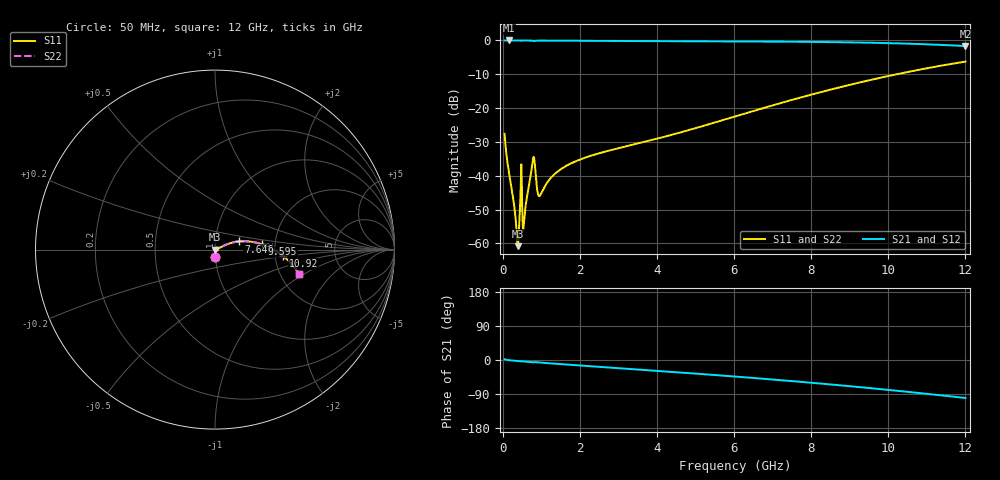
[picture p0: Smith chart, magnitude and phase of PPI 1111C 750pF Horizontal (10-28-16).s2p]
# MHz S MA R 50
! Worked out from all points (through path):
!   1601 points, 50 MHz to 12 GHz, reference 50 ohm
!   highest |S21| = 0.00 dB at 154.6 MHz (marker M1); lowest = -1.7 dB at 12 GHz (marker M2)
!   group delay of S21, straight-line fit = 22.7 ps
!   lowest |S11| = -60.8 dB at 393.6 MHz (marker M3), VSWR 1.00, Z = 50.1 - j0.0133 ohm
!   |S11| at or under -10 dB: start of sweep to 10.22 GHz
!   |S22| runs from -60.8 to -6.3 dB; largest |S21 - S12| = 0
!   S11 on the Smith chart (normalised r, x): 50 MHz: 1.00, -0.08; 7.646 GHz: 1.30, +0.12; 9.595 GHz: 1.71, +0.11; 10.92 GHz: 2.21, -0.18; 12 GHz: 2.53, -0.89
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50  0.04163 -87.5  0.9988 2.0  0.9988 2.0  0.04163 -87.5
154.5625  0.01199 -88.1  0.9995 -0.4  0.9995 -0.4  0.01199 -88.1
274.0625  0.004582 -83.9  0.9994 -1.6  0.9994 -1.6  0.004582 -83.9
356.2188  0.001653 -64.2  0.9992 -2.4  0.9992 -2.4  0.001653 -64.2
393.5625  0.0009092 -8.4  0.9991 -2.7  0.9991 -2.7  0.0009092 -8.4
468.25  0.00666 56.9  0.9967 -3.6  0.9967 -3.6  0.00666 56.9
520.5312  0.001777 -22.1  0.9983 -3.6  0.9983 -3.6  0.001777 -22.1
572.8125  0.00282 52.3  0.9984 -4.1  0.9984 -4.1  0.00282 52.3
781.9375  0.01696 38.0  0.9877 -6.1  0.9877 -6.1  0.01696 38.0
826.75  0.01631 -7.6  0.9836 -5.7  0.9836 -5.7  0.01631 -7.6
916.375  0.005339 -3.8  0.9946 -6.3  0.9946 -6.3  0.005339 -3.8
968.6562  0.005106 19.4  0.9954 -6.8  0.9954 -6.8  0.005106 19.4
1379.438  0.01098 41.9  0.9931 -10.0  0.9931 -10.0  0.01098 41.9
2044.156  0.01769 32.3  0.9877 -14.7  0.9877 -14.7  0.01769 32.3
4038.312  0.0357 22.3  0.9769 -28.8  0.9769 -28.8  0.0357 22.3
6025  0.07517 23.8  0.9684 -43.6  0.9684 -43.6  0.07517 23.8
7645.719  0.1392 19.0  0.9565 -56.9  0.9565 -56.9  0.1392 19.0
8019.156  0.159 17.1  0.9523 -60.1  0.9523 -60.1  0.159 17.1
9595.062  0.2648 6.3  0.924 -74.8  0.924 -74.8  0.2648 6.3
10013.31  0.2989 2.9  0.9125 -79.0  0.9125 -79.0  0.2989 2.9
10924.5  0.3806 -5.3  0.8798 -88.4  0.8798 -88.4  0.3806 -5.3
12000  0.4864 -16.0  0.8255 -100.2  0.8255 -100.2  0.4864 -16.0
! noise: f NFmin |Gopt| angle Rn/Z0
50  0.000383  0.8696  0.3678  0.0006323
1372  0.009288  0.8545  9.417  0.01354
2701  0.02023  0.8697  18.41  0.03256
4031  0.02862  0.8666  27.15  0.04357
5360  0.03554  0.8627  35.56  0.05035
6682  0.04179  0.8609  43.52  0.05557
8012  0.04789  0.8617  51.08  0.06052
9341  0.05412  0.865  58.17  0.06585
1.067e+04  0.06072  0.8703  64.79  0.07202
1.2e+04  0.06795  0.8772  70.95  0.07949
